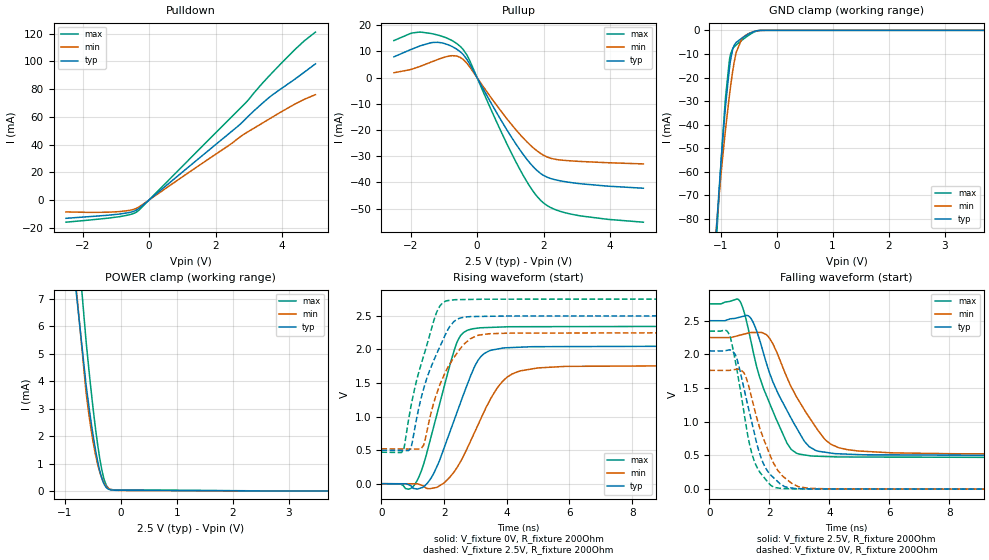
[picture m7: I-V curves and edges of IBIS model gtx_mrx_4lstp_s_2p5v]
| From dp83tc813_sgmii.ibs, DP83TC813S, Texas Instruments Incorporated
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| gtx_mrx_4lstp_s_2p5v
[Model]   gtx_mrx_4lstp_s_2p5v
Model_type   I/O
Polarity   Non-Inverting
Enable   Active-Low
Vinl = 0.7
Vinh = 1.7
Vmeas = 1.25
Vref = 1.25
Cref = 2pF
Rref = 100000
|   typ   min   max
C_comp   2.97pF   2.92pF   3pF
[Voltage Range]   2.5   2.25   2.75
[Temperature Range]   27   150   -40
[Pullup Reference]   2.5   2.25   2.75
[Pulldown Reference]   -0   0   -0
[Power Clamp Reference]   2.5   2.25   2.75
[GND Clamp Reference]   0   0   0
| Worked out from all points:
|   slope of the pulldown table from 0 to 0.375 V, typ, clamps not added: 49.7 ohm
|   slope of the pullup table from 0 to 0.375 V, typ, clamps not added: 43.5 ohm
|   GND clamp passes 1 mA (typ) near -0.45 V on its own axis
|   POWER clamp passes 1 mA (typ) near -0.40 V on its own axis
|   falling waveform, V_fixture 2.5V, R_fixture 200Ohm: 20-80 % time 1.17ns typ, 1.27ns min, 1.01ns max; typ from 2.5 V to 0.498 V
|   rising waveform, V_fixture 0V, R_fixture 200Ohm: 20-80 % time 973ps typ, 1.12ns min, 797ps max; typ from 0 V to 2.05 V
|   rising waveform, V_fixture 2.5V, R_fixture 200Ohm: 20-80 % time 829ps typ, 859ps min, 733ps max; typ from 0.498 V to 2.5 V
|   falling waveform, V_fixture 0V, R_fixture 200Ohm: 20-80 % time 693ps typ, 804ps min, 584ps max; typ from 2.05 V to 0 V
[Pulldown]
|   Voltage   I(typ)   I(min)   I(max)
-2.5V     -13.29mA   -8.687mA   -16.1mA
-925mV    -10.31mA   -8.492mA   -12.22mA
-512.5mV  -8.603mA   -7.139mA   -10.18mA
-347.5mV  -6.835mA   -5.631mA   -8.211mA
2.638V    52.57mA    43.69mA    63.75mA
2.885V    58.13mA    47.96mA    69.7mA
3.462V    71.02mA    56.29mA    85.76mA
3.958V    80.11mA    63.41mA    98.27mA
4.633V    91.66mA    72.28mA    114.2mA
5V        98.27mA    76.01mA    121.2mA
[GND Clamp]
|   Voltage   I(typ)   I(min)   I(max)
-2.5V     -648.4mA   -555.8mA   -723.6mA
-1.097V   -92.72mA   -89.85mA   -98.54mA
-1.03V    -68.88mA   -71.01mA   -71.09mA
-962.5mV  -46.81mA   -53.8mA    -45.43mA
-917.5mV  -33.73mA   -43.36mA   -30.37mA
-835mV    -14.9mA    -26.33mA   -11.67mA
-782.5mV  -8.005mA   -17.22mA   -7.74mA
-722.5mV  -5.155mA   -9.439mA   -6.239mA
-617.5mV  -3.266mA   -3.489mA   -4.19mA
-497.5mV  -1.539mA   -1.362mA   -2.076mA
-265mV    -17.6uA    -39uA      -18.83uA
5V        0A         0A         0A
[Pullup]
|   Voltage   I(typ)   I(min)   I(max)
-2.5V     7.944mA    1.866mA    14.16mA
-1.938V   11mA       3.316mA    17.07mA
-1.315V   13.45mA    6.279mA    16.67mA
-752.5mV  11.89mA    8.383mA    14.16mA
-460mV    9.358mA    7.341mA    11.34mA
-257.5mV  5.988mA    4.704mA    7.488mA
642.5mV   -14.55mA   -11.48mA   -18.41mA
1.272V    -27.27mA   -21.43mA   -34.67mA
1.677V    -33.87mA   -26.64mA   -43.23mA
2.007V    -37.38mA   -29.68mA   -47.93mA
2.953V    -40.27mA   -31.88mA   -52.42mA
5V        -42.22mA   -32.93mA   -55.18mA
[POWER Clamp]
|   Voltage   I(typ)   I(min)   I(max)
-2.5V     111.6mA    76.29mA    155.1mA
-1.06V    12.33mA    13.14mA    16.14mA
-617.5mV  3.849mA    3.558mA    5.431mA
-557.5mV  2.922mA    2.624mA    4.207mA
-505mV    2.182mA    1.927mA    3.214mA
-445mV    1.436mA    1.271mA    2.191mA
-392.5mV  892.8uA    818.2uA    1.42mA
-347.5mV  528.8uA    520.2uA    876.1uA
-302.5mV  272.9uA    303.6uA    464.8uA
-257.5mV  124.4uA    163.1uA    204.9uA
-212.5mV  57.82uA    83.72uA    84.66uA
5V        0A         0A         0A
[Ramp]
R_load = 200
|   typ   min   max
dV/dt_r   1.2299/9.67872e-10   1.05633/1.11999e-09   1.40654/7.94538e-10
dV/dt_f   1.2005/1.16325e-09   1.03762/1.26579e-09   1.36792/9.99845e-10
[Falling Waveform]
V_fixture = 2.5V
V_fixture_min = 2.25V
V_fixture_max = 2.75V
R_fixture = 200Ohm
C_fixture = 0F
|   Time   V(typ)   V(min)   V(max)
0s        2.499V     2.249V     2.749V
1.027ns   2.553V     2.285V     2.783V
1.394ns   2.528V     2.323V     2.179V
1.923ns   1.839V     2.283V     1.367V
2.592ns   1.165V     1.654V     680.7mV
2.907ns   909.6mV    1.369V     533.5mV
3.329ns   630.3mV    1.066V     497.3mV
3.844ns   548.9mV    743.1mV    484.9mV
4.575ns   520.1mV    588.4mV    477.4mV
12ns      498.3mV    519.8mV    469.1mV
[Rising Waveform]
V_fixture = 0V
V_fixture_min = 0V
V_fixture_max = 0V
R_fixture = 200Ohm
C_fixture = 0F
|   Time   V(typ)   V(min)   V(max)
0s        117.6uV    205.5uV    101.9uV
856ps     -12.44mV   -872.9uV   -81.4mV
1.124ns   -77.81mV   -1.211mV   34.47mV
1.679ns   160.8mV    -62.55mV   868.6mV
2.349ns   982.2mV    196.9mV    2.026V
2.735ns   1.471V     525mV      2.283V
3.294ns   1.943V     1.09V      2.324V
3.844ns   2.016V     1.514V     2.333V
4.403ns   2.032V     1.676V     2.337V
12ns      2.05V      1.761V     2.344V
[Rising Waveform]
V_fixture = 2.5V
V_fixture_min = 2.25V
V_fixture_max = 2.75V
R_fixture = 200Ohm
C_fixture = 0F
|   Time   V(typ)   V(min)   V(max)
0s        498.3mV    519.8mV    469.1mV
704.9ps   494mV      516.8mV    505.1mV
934.1ps   532.6mV    515.9mV    1.132V
1.346ns   1.412V     575.3mV    1.902V
1.75ns    1.921V     1.324V     2.538V
2.037ns   2.216V     1.658V     2.716V
2.32ns    2.417V     1.883V     2.738V
2.823ns   2.487V     2.155V     2.743V
3.447ns   2.493V     2.233V     2.747V
12ns      2.499V     2.249V     2.749V
[Falling Waveform]
|Gnd
V_fixture = 0V
V_fixture_min = 0V
V_fixture_max = 0V
R_fixture = 200Ohm
C_fixture = 0F
|   Time   V(typ)   V(min)   V(max)
0s        2.051V     1.762V     2.345V
601.4ps   2.06V      1.761V     2.34V
869ps     1.993V     1.776V     1.891V
1.153ns   1.497V     1.726V     1.142V
1.432ns   958.7mV    1.318V     505.6mV
1.737ns   449.6mV    834.7mV    220.4mV
2.144ns   169.3mV    384.5mV    31.89mV
2.749ns   16.96mV    85.64mV    5.974mV
3.321ns   5.147mV    12.23mV    2.683mV
12ns      117.5uV    206.6uV    101.7uV
